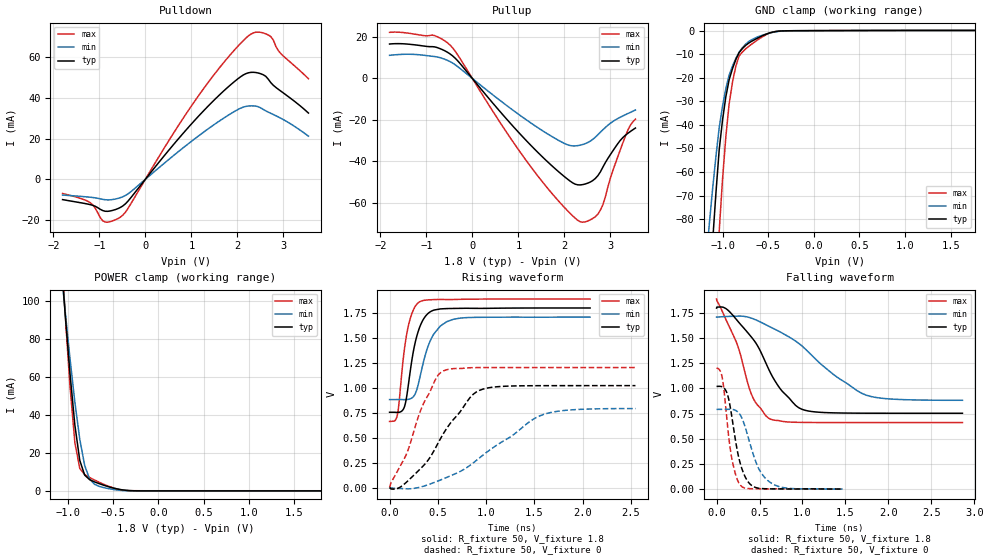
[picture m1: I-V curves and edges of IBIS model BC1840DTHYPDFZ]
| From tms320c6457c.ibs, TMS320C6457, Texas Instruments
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|   Component BC1840DTHYPDFZ
|BUFFER OPERATING IN WEAK PULLDOWN MODE WITH +/- 5% VDDS
|   Model Cell BC1840DTHYPDFZ
[Model]   BC1840DTHYPDFZ
Model_type   I/O
Polarity   Non-Inverting
Enable   Active-Low
Vinl =  0.63
Vinh =  1.17
Cref =  15pF
Rref =  100.00M
Vref =  0V
Vmeas =  0.9
C_comp   1.427611p   1.198581p   1.770817p
[Model Spec]
Vinl   0.63   0.5985   0.6615
Vinh   1.17   1.1115   1.2285
[Temperature Range]   25   125   -40
[Voltage Range]   1.8   1.71   1.89
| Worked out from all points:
|   slope of the pulldown table from 0 to 0.27 V, typ, clamps not added: 35.3 ohm
|   slope of the pullup table from 0 to 0.27 V, typ, clamps not added: 37.2 ohm
|   GND clamp passes 1 mA (typ) near -0.49 V on its own axis
|   POWER clamp passes 1 mA (typ) near -0.45 V on its own axis
|   rising waveform, R_fixture 50, V_fixture 1.8: 20-80 % time 121ps typ, 161ps min, 96.4ps max; typ from 0.754 V to 1.8 V
|   rising waveform, R_fixture 50, V_fixture 0: 20-80 % time 436ps typ, 689ps min, 295ps max; typ from 0 V to 1.02 V
|   falling waveform, R_fixture 50, V_fixture 1.8: 20-80 % time 448ps typ, 744ps min, 293ps max; typ from 1.8 V to 0.754 V
|   falling waveform, R_fixture 50, V_fixture 0: 20-80 % time 135ps typ, 194ps min, 104ps max; typ from 1.02 V to 0.002 V
[Pulldown]
|   voltage   I(typ)   I(min)   I(max)
-1.8V     -9.973mA   -7.74mA    -6.977mA
-1.2V     -12.43mA   -8.798mA   -11.45mA
-872.7mV  -15.69mA   -10.03mA   -21mA
-490.9mV  -13.1mA    -8.568mA   -17.62mA
600mV     16.72mA    11.42mA    22.21mA
1.2V      32.04mA    22.03mA    42.42mA
2.018V    49.45mA    34.33mA    65.47mA
2.345V    52.52mA    36.03mA    71.85mA
2.564V    51.3mA     34.29mA    71.83mA
2.727V    47.43mA    32.37mA    70.04mA
2.945V    43.27mA    29.96mA    61.7mA
3.545V    32.51mA    21.19mA    49.34mA
[Pullup]
|   voltage   I(typ)   I(min)   I(max)
-1.8V     16.61mA    11.16mA    22.24mA
-872.7mV  15.35mA    10.7mA     20.95mA
-490.9mV  11.93mA    8.207mA    16.23mA
1.2V      -30.58mA   -20.35mA   -40.43mA
2.018V    -47.62mA   -31.49mA   -62.56mA
2.345V    -51.31mA   -32.14mA   -69.06mA
2.618V    -49.2mA    -29.35mA   -67.48mA
2.782V    -45.07mA   -25.91mA   -63.52mA
3.109V    -33.1mA    -19.97mA   -40.94mA
3.327V    -27.37mA   -17.47mA   -27.8mA
3.436V    -25.53mA   -16.32mA   -22.48mA
3.545V    -23.89mA   -15.19mA   -19.61mA
[GND_clamp]
|   voltage   I(typ)   I(min)   I(max)
-1.8V     -628.4mA   -433.3mA   -1A
-1.145V   -112.8mA   -82.32mA   -190.2mA
-1.109V   -89.95mA   -67.31mA   -152.1mA
-1.073V   -69.17mA   -53.57mA   -117.1mA
-1.036V   -50.48mA   -41.1mA    -85.11mA
-963.6mV  -28.05mA   -24.6mA    -45.07mA
-927.3mV  -20.79mA   -18.8mA    -31.03mA
-890.9mV  -16.13mA   -15.03mA   -21.88mA
-818.2mV  -9.298mA   -9.115mA   -10.72mA
-709.1mV  -5.166mA   -4.488mA   -6.537mA
-381.8mV  -183uA     -282.8uA   -155.6uA
1.764V    90uA       54.73uA    144.6uA
[POWER_clamp]
|   voltage   I(typ)   I(min)   I(max)
-1.8V     632.9mA    511.7mA    764.9mA
-1.055V   105.5mA    104.1mA    108.5mA
-1.036V   93.96mA    95.21mA    94.18mA
-981.8mV  61.95mA    69.81mA    55.29mA
-927.3mV  34.63mA    46.66mA    25.43mA
-872.7mV  16.07mA    27.16mA    11.89mA
-818.2mV  8.339mA    13.39mA    8.624mA
-763.6mV  5.979mA    6.278mA    7.106mA
-709.1mV  4.79mA     3.529mA    5.787mA
-490.9mV  1.445mA    754.2uA    1.49mA
-327.3mV  239.5uA    110.1uA    248uA
1.8V      90.13uA    54.57uA    145.3uA
[Ramp]
| variable   typ   min   max
dV/dt_f  0.6332775/0.4540206n  0.5024231/0.7581118n  0.7424777/0.2963035n
dV/dt_r  0.6220983/0.4475145n  0.4832185/0.7087564n  0.7322463/0.3015353n
R_load = 50
[Rising Waveform]
R_fixture = 50
V_fixture = 1.8
V_fixture_min = 1.71
V_fixture_max = 1.89
|   time   V(typ)   V(min)   V(max)
0s        753.7mV    880.8mV    661.4mV
80ps      752.1mV    881.1mV    722.6mV
154ps     808.3mV    880.1mV    1.387V
220ps     1.204V     890.9mV    1.71V
266ps     1.454V     938.8mV    1.815V
312ps     1.605V     1.093V     1.86V
374ps     1.718V     1.34V      1.877V
428ps     1.764V     1.483V     1.881V
594ps     1.792V     1.662V     1.882V
2.078ns   1.798V     1.707V     1.887V
[Rising Waveform]
R_fixture = 50
V_fixture = 0
V_fixture_min = 0
V_fixture_max = 0
|   time   V(typ)   V(min)   V(max)
0s        89.2nV     175.9nV    34.46nV
84ps      -8.915mV   -8.458mV   168.6mV
190ps     66.66mV    -13.07mV   370.9mV
330ps     198.3mV    7.271mV    792.1mV
488ps     418.3mV    60.38mV    1.104V
558ps     540.3mV    87.47mV    1.168V
834ps     901mV      222.6mV    1.2V
994ps     992.4mV    344.3mV    1.202V
1.6ns     1.02V      733.5mV    1.202V
2.548ns   1.02V      790.6mV    1.202V
[Falling Waveform]
R_fixture = 50
V_fixture = 1.8
V_fixture_min = 1.71
V_fixture_max = 1.89
|   time   V(typ)   V(min)   V(max)
0s        1.798V     1.709V     1.887V
108ps     1.793V     1.714V     1.686V
248ps     1.667V     1.718V     1.42V
422ps     1.493V     1.693V     910.9mV
614ps     1.178V     1.615V     701.4mV
772ps     965.1mV    1.546V     672.6mV
1.034ns   782.3mV    1.391V     662.6mV
1.37ns    757.6mV    1.133V     661.5mV
1.744ns   754.3mV    932.8mV    661.4mV
2.862ns   753.7mV    882.6mV    661.4mV
[Falling Waveform]
R_fixture = 50
V_fixture = 0
V_fixture_min = 0
V_fixture_max = 0
|   time   V(typ)   V(min)   V(max)
0s        1.02V      792.3mV    1.202V
68ps      1.016V     792.3mV    1.097V
126ps     942.3mV    792.3mV    645.4mV
156ps     830.7mV    793.1mV    420.8mV
192ps     639.4mV    791mV      245.4mV
286ps     225.9mV    720.9mV    31.64mV
372ps     67.75mV    503.8mV    6.043mV
484ps     10.39mV    216.3mV    3.651mV
636ps     3.228mV    60.24mV    2.484mV
1.466ns   1.69mV     1.716mV    144.4uV
